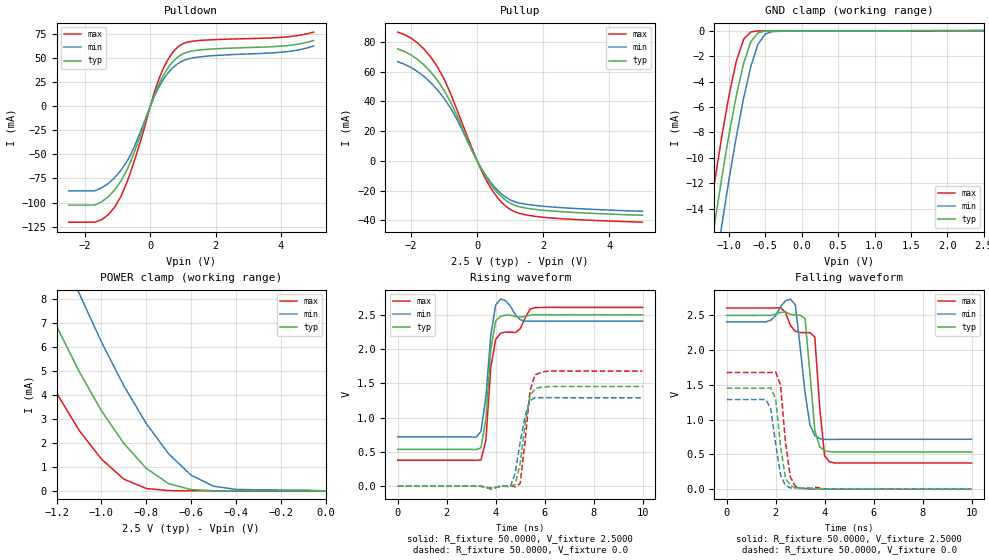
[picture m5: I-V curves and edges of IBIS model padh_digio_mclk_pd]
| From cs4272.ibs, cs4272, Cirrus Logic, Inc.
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|   Model mclkp
[Model]  padh_digio_mclk_pd
Model_type I/O
Polarity   Non-Inverting
Enable   Active-High
Vinl =   0.8000V
Vinh =   2.0000V
C_comp   5.0000pF   5.0000pF   5.0000pF
[Temperature Range]   25.0000   85.0000   -40.0000
[Voltage Range]   2.5000V   2.2500V   2.7500V
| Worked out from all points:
|   slope of the pulldown table from 0 to 0.375 V, typ, clamps not added: 12.4 ohm
|   slope of the pullup table from 0 to 0.375 V, typ, clamps not added: 25.7 ohm
|   GND clamp passes 1 mA (typ) near -0.71 V on its own axis
|   POWER clamp passes 1 mA (typ) near -0.81 V on its own axis
|   rising waveform, R_fixture 50.0000, V_fixture 2.5000: 20-80 % time 276ps typ, 270ps min, 415ps max; typ from 0.535 V to 2.5 V
|   rising waveform, R_fixture 50.0000, V_fixture 0.0: 20-80 % time 351ps typ, 380ps min, 292ps max; typ from 0 V to 1.45 V
|   falling waveform, R_fixture 50.0000, V_fixture 2.5000: 20-80 % time 290ps typ, 352ps min, 295ps max; typ from 2.5 V to 0.535 V
|   falling waveform, R_fixture 50.0000, V_fixture 0.0: 20-80 % time 304ps typ, 326ps min, 298ps max; typ from 1.45 V to 0 V
[Pulldown]
|Voltage   I(typ)   I(min)   I(max)
-2.5V     -102.6mA   -87.82mA   -120.3mA
-1.7V     -102.6mA   -87.82mA   -120.3mA
-1.3V     -94.3mA    -80.5mA    -112.9mA
-1.1V     -87.15mA   -74.4mA    -105mA
-900mV    -77.64mA   -66.5mA    -93.5mA
-600mV    -57.17mA   -50.03mA   -67.82mA
300mV     25.49mA    22.02mA    31.38mA
600mV     42.28mA    36.63mA    51.46mA
900mV     52.12mA    45.2mA     62.7mA
1.5V      57.98mA    50.84mA    67.85mA
4V        62.02mA    55.7mA     71.09mA
5V        67.75mA    62.13mA    76.56mA
[Pullup]
|Voltage   I(typ)   I(min)   I(max)
-2.4V     75.35mA    66.72mA    86.65mA
-1.8V     68.25mA    60.06mA    79.34mA
-1.2V     54.2mA     47.74mA    63.26mA
-1V       47.52mA    42.08mA    55.15mA
-600mV    29.95mA    27.57mA    33.85mA
-100mV    4.665mA    4.31mA     5.4mA
200mV     -8.394mA   -7.73mA    -9.741mA
500mV     -18.4mA    -16.95mA   -21.23mA
900mV     -27.12mA   -24.98mA   -31.11mA
1.3V      -31.04mA   -28.53mA   -35.48mA
1.9V      -33.02mA   -30.34mA   -37.73mA
5V        -36.63mA   -33.94mA   -41.29mA
[GND_clamp]
|Voltage   I(typ)   I(min)   I(max)
-2.5V     -71.97mA   -75.47mA   -70.88mA
-1.3V     -19.2mA    -23.2mA    -15.95mA
-1.2V     -15.29mA   -19.19mA   -11.99mA
-1.1V     -11.58mA   -15.35mA   -8.339mA
-1V       -8.151mA   -11.69mA   -5.092mA
-900mV    -5.126mA   -8.35mA    -2.408mA
-800mV    -2.58mA    -5.322mA   -669.6uA
-700mV    -857.9uA   -2.786mA   -83.92uA
-600mV    -149.6uA   -1.035mA   -8.308uA
-500mV    -15.48uA   -242.8uA   -3.519uA
-400mV    -2.927uA   -59.61uA   -2.67uA
2.5V      3.356uA    40.4uA     4.32uA
[POWER_clamp]
|Voltage   I(typ)   I(min)   I(max)
-2.5V     42.45mA    48.26mA    38.67mA
-1.4V     11.23mA    15.42mA    7.976mA
-1.3V     8.974mA    12.89mA    5.923mA
-1.2V     6.887mA    10.5mA     4.097mA
-1.1V     5.001mA    8.267mA    2.54mA
-1V       3.348mA    6.22mA     1.329mA
-900mV    1.985mA    4.389mA    491.5uA
-800mV    942.6uA    2.813mA    100.1uA
-700mV    302.3uA    1.544mA    13.81uA
-600mV    55.15uA    654.1uA    4.877uA
-400mV    3.685uA    64.83uA    4.327uA
0V        0A         0A         0A
[Ramp]
| variable   typ   min   max
dV/dt_r  0.8718/0.3281n   0.6714/0.4192n   1.1028/0.2379n
dV/dt_f  1.1783/0.2423n   0.9585/0.3256n   1.3993/0.1786n
R_load = 50.0000
[Rising Waveform]
R_fixture= 50.0000
V_fixture= 2.5000
V_fixture_min= 2.7500
V_fixture_max= 2.2500
|time   V(typ)   V(min)   V(max)
0s        535.2mV    717.8mV    376.7mV
3.2ns     532.9mV    714.9mV    375.3mV
3.4ns     558.4mV    798.5mV    381.9mV
3.6ns     969.7mV    1.301V     667.1mV
3.8ns     1.988V     2.195V     1.73V
4ns       2.409V     2.642V     2.14V
4.2ns     2.476V     2.728V     2.23V
4.8ns     2.474V     2.502V     2.24V
5.6ns     2.5V       2.406V     2.604V
10ns      2.499V     2.406V     2.606V
[Rising Waveform]
R_fixture= 50.0000
V_fixture= 0.0
|time   V(typ)   V(min)   V(max)
0s        0V         230.1uV    0V
3.8ns     -37.84mV   -25.43mV   -44.82mV
4.6ns     -5.028mV   -11.82mV   412.5uV
4.8ns     26.99mV    189.8mV    -9.123mV
5ns       325.1mV    634mV      35.53mV
5.2ns     897.4mV    1.018V     649.4mV
5.4ns     1.311V     1.247V     1.379V
5.6ns     1.421V     1.288V     1.621V
6.2ns     1.452V     1.29V      1.677V
10ns      1.453V     1.289V     1.678V
[Falling Waveform]
R_fixture= 50.0000
V_fixture= 2.5000
V_fixture_min= 2.7500
V_fixture_max= 2.2500
|time   V(typ)   V(min)   V(max)
0s        2.499V     2.406V     2.606V
1.6ns     2.499V     2.407V     2.606V
2.2ns     2.541V     2.623V     2.614V
2.8ns     2.503V     2.656V     2.27V
3.2ns     2.454V     1.393V     2.251V
3.6ns     841.4mV    770.7mV    2.188V
3.8ns     611mV      726.7mV    1.17V
4ns       550mV      716mV      477.6mV
4.2ns     540.6mV    714.9mV    393.4mV
10ns      535.2mV    717.4mV    376.7mV
[Falling Waveform]
R_fixture= 50.0000
V_fixture= 0.0
|time   V(typ)   V(min)   V(max)
0s        1.453V     1.289V     1.678V
1.6ns     1.453V     1.288V     1.678V
1.8ns     1.458V     1.156V     1.678V
2ns       1.299V     655.4mV    1.684V
2.2ns     618.5mV    204.4mV    1.496V
2.4ns     162mV      51.9mV     679.3mV
2.6ns     56.23mV    18.65mV    173.8mV
2.8ns     17.05mV    19.98mV    44.65mV
3.4ns     18.41mV    3.014mV    3.618mV
10ns      2.227uV    0V         -2.196uV
